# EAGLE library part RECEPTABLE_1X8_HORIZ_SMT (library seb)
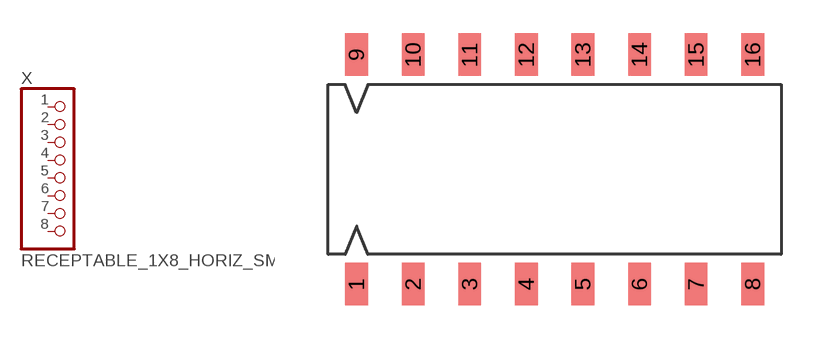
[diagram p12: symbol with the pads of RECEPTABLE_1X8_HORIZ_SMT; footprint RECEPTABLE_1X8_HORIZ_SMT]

Designator prefix X

## RECEPTABLE_1X8_HORIZ_SMT  [RECEPTABLE_1X8_HORIZ_SMT]
1  1  pwr
2  2  pwr
3  3  pwr
4  4  pwr
5  5  pwr
6  6  pwr
7  7  pwr
8  8  pwr
9  1  pwr
10  2  pwr
11  3  pwr
12  4  pwr
13  5  pwr
14  6  pwr
15  7  pwr
16  8  pwr

## Footprint RECEPTABLE_1X8_HORIZ_SMT (pad centres in mm)
smd 1.016 x 1.905: 1 -8.89,-5.144; 2 -6.35,-5.144; 3 -3.81,-5.144; 4 -1.27,-5.144; 5 1.27,-5.144; 6 3.81,-5.144; 7 6.35,-5.144; 8 8.89,-5.144; 9 -8.89,5.144; 10 -6.35,5.144; 11 -3.81,5.144; 12 -1.27,5.144; 13 1.27,5.144; 14 3.81,5.144; 15 6.35,5.144; 16 8.89,5.144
